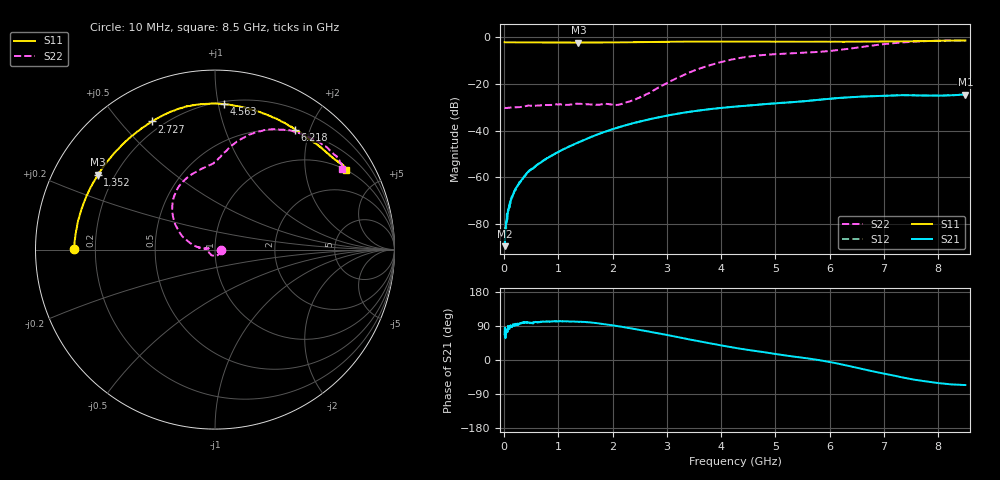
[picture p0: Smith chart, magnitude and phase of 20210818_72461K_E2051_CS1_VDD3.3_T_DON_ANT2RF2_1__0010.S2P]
!Agilent Technologies,E5071C,MY46417908,A.11.23
!Date: Wed Aug 18 14:26:36 2021
!Data & Calibration Information:
!Freq	S11:SOLT2(ON)	S21:SOLT2(ON)	S12:SOLT2(ON)	S22:SOLT2(ON)
!PortZ  Port1:50+j0  Port2:50+j0
!Above PortZ is port z conversion or system Z0 setting when saving the data.
!When reading, reference impedance value at option line is always used.
# Hz S dB R 50
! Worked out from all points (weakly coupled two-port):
!   1601 points, 10 MHz to 8.5 GHz, reference 50 ohm
!   highest |S21| = -24.55 dB at 8.5 GHz (marker M1); lowest = -89.6 dB at 15.31 MHz (marker M2)
!   lowest |S11| = -2.2 dB at 1.368 GHz (marker M3), VSWR 7.81, Z = 6.94 + j14.4 ohm
!   |S11| at or under -10 dB: nowhere
!   |S22| runs from -30.4 to -1.4 dB; largest |S21 - S12| = 0.00028
!   S11 on the Smith chart (normalised r, x): 10 MHz: 0.12, +0.00; 1.352 GHz: 0.14, +0.28; 2.727 GHz: 0.16, +0.61; 4.563 GHz: 0.22, +1.04; 6.218 GHz: 0.47, +1.77; 8.5 GHz: 1.00, +3.28
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1e7  -2.08 179.7  -88.60 67.8  -88.89 62.3  -30.13 -2.4
1.530625e7  -2.09 179.6  -89.57 85.6  -85.37 42.0  -30.18 -3.3
5.775625e7  -2.12 178.7  -78.32 79.0  -77.11 76.3  -30.29 -7.3
1.055125e8  -2.12 177.6  -71.03 89.7  -71.73 86.5  -30.16 -12.2
1.744938e8  -2.13 176.0  -66.98 91.3  -66.60 91.7  -29.99 -18.9
2.540875e8  -2.14 174.1  -63.37 95.3  -63.50 95.2  -29.98 -28.9
4.238875e8  -2.16 170.2  -58.14 99.0  -58.21 99.2  -29.37 -53.0
7.741e8  -2.19 161.9  -52.09 101.5  -52.15 101.8  -29.04 -95.6
1.352481e9  -2.22 147.7  -45.24 101.2  -45.26 101.0  -28.47 -158.2
1.3684e9  -2.24 147.4  -45.05 100.7  -45.15 101.0  -28.48 -159.4
1.426769e9  -2.22 145.8  -44.50 100.7  -44.50 100.5  -28.55 -163.9
2.116581e9  -2.14 128.9  -38.56 88.9  -38.57 88.7  -28.87 168.3
2.7268e9  -1.99 116.1  -34.89 73.2  -34.89 73.4  -23.12 174.0
2.843538e9  -1.96 114.2  -34.34 70.2  -34.34 70.2  -21.53 173.0
3.4909e9  -1.82 103.8  -31.71 52.2  -31.69 52.2  -14.32 158.5
4.255e9  -1.79 91.8  -29.72 32.1  -29.73 32.1  -9.24 133.4
4.562762e9  -1.81 86.4  -29.14 25.4  -29.14 25.3  -8.10 122.8
5.671769e9  -1.88 65.0  -27.08 2.7  -27.07 2.8  -6.44 92.2
6.218312e9  -1.90 56.3  -25.92 -11.5  -25.94 -11.5  -5.29 84.5
7.088538e9  -1.75 45.3  -24.94 -38.4  -24.97 -38.6  -2.68 65.6
7.921619e9  -1.51 36.0  -25.00 -59.3  -24.98 -59.3  -1.48 42.6
8.5e9  -1.37 31.4  -24.55 -66.1  -24.57 -66.3  -1.53 32.3
